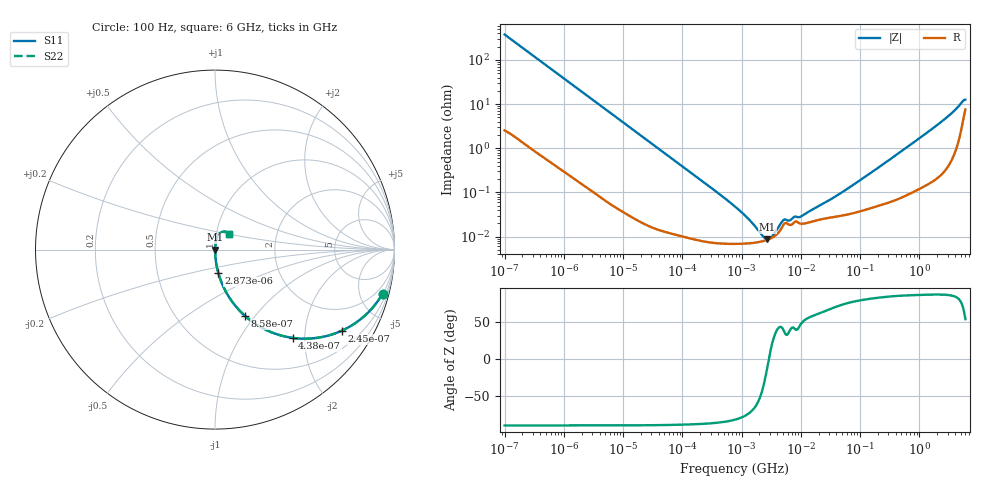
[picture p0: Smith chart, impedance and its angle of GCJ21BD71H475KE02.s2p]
!Murata Part Number: GCJ21BD71H475KE02
!These Parameters are Measured in Series Mode Connection
!Data Generated on Mar 13, 2026
!  o--ll--o
!Port1  Port2
!  o------o
!Operation Temp=25[degC], DC Bias Voltage=0[V]
!Freq. Start=100[Hz] Stop=6[GHz] 401[Steps]
# Hz S RI R 50
!Freq.(Hz) S11(Real) S11(Imag) S21(Real) S21(Imag) S12(Real) S12(Imag) S22(Real) S22(Imag)
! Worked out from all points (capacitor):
!   401 points, 100 Hz to 6 GHz, reference 50 ohm
!   read as one part in series: C = 4.19 uF near 109 Hz
!   lowest |Z| = 8.64 mohm at 2.714 MHz (marker M1)
!   series resonance near 2.893 MHz, so ESL is about 720 pH
!   S11 on the Smith chart (normalised r, x): 100 Hz: 1.05, -7.58; 245 Hz: 1.02, -3.11; 438 Hz: 1.01, -1.74; 858 Hz: 1.01, -0.89; 2.873 kHz: 1.00, -0.27; 6 GHz: 1.15, +0.20
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100  0.9335 -0.2458  0.0665 0.2458  0.0665 0.2458  0.9335 -0.2458
164  0.8419 -0.3613  0.1581 0.3613  0.1581 0.3613  0.8419 -0.3613
245  0.7063 -0.4519  0.2937 0.4519  0.2937 0.4519  0.7063 -0.4519
438  0.4322 -0.4917  0.5678 0.4917  0.5678 0.4917  0.4322 -0.4917
858  0.1682 -0.3703  0.8318 0.3703  0.8318 0.3703  0.1682 -0.3703
2008  0.0368 -0.1842  0.9632 0.1842  0.9632 0.1842  0.0368 -0.1842
2873  0.0187 -0.1315  0.9813 0.1315  0.9813 0.1315  0.0187 -0.1315
8416  0.00253 -0.0459  0.9975 0.0459  0.9975 0.0459  0.00253 -0.0459
40335  0.000234 -0.00967  0.9998 0.00967  0.9998 0.00967  0.000234 -0.00967
774597  6.85e-05 -0.000475  0.9999 0.000475  0.9999 0.000475  6.85e-05 -0.000475
1325623  7.04e-05 -0.000236  0.9999 0.000236  0.9999 0.000236  7.04e-05 -0.000236
2169299  7.75e-05 -8.04e-05  0.9999 8.04e-05  0.9999 8.04e-05  7.75e-05 -8.04e-05
2713602  8.45e-05 -1.78e-05  0.9999 1.78e-05  0.9999 1.78e-05  8.45e-05 -1.78e-05
3394479  9.7e-05 4.51e-05  0.9999 -4.51e-05  0.9999 -4.51e-05  9.7e-05 4.51e-05
5079039  0.000184 0.000149  0.9998 -0.000149  0.9998 -0.000149  0.000184 0.000149
9941735  0.000196 0.000205  0.9998 -0.000205  0.9998 -0.000205  0.000196 0.000205
1.555665e7  0.00022 0.000343  0.9998 -0.000343  0.9998 -0.000343  0.00022 0.000343
4.983056e7  0.0003 0.000965  0.9997 -0.000965  0.9997 -0.000965  0.0003 0.000965
3.124326e8  0.000625 0.00545  0.9994 -0.00545  0.9994 -0.00545  0.000625 0.00545
3.505958e9  0.00907 0.0611  0.9909 -0.0611  0.9909 -0.0611  0.00907 0.0611
5.245841e9  0.0406 0.0986  0.9594 -0.0986  0.9594 -0.0986  0.0406 0.0986
6e9  0.0784 0.0871  0.9216 -0.0871  0.9216 -0.0871  0.0784 0.0871
